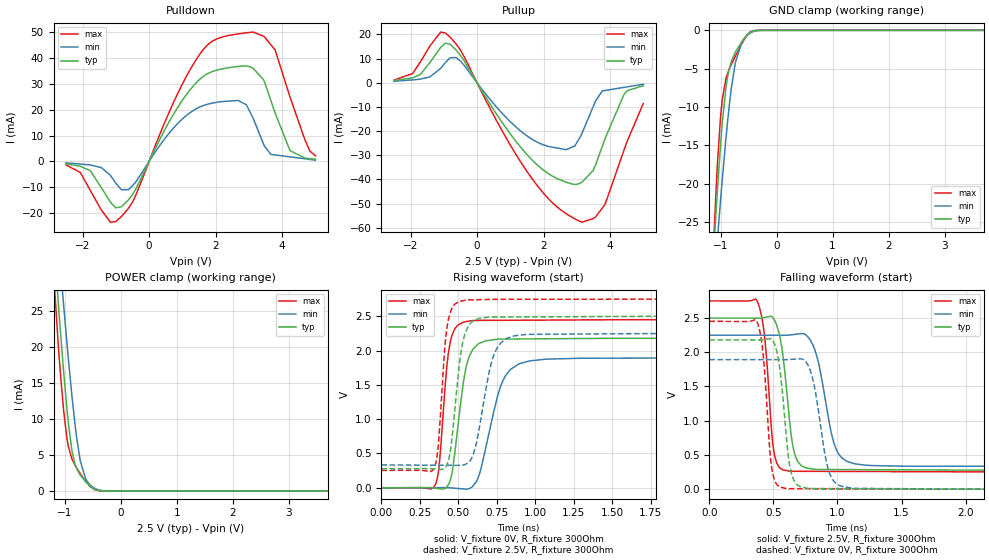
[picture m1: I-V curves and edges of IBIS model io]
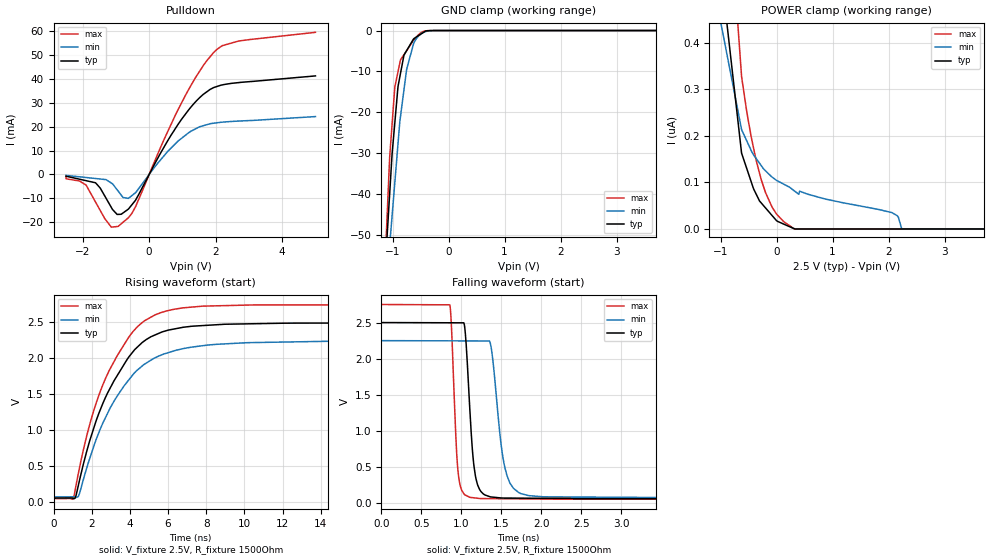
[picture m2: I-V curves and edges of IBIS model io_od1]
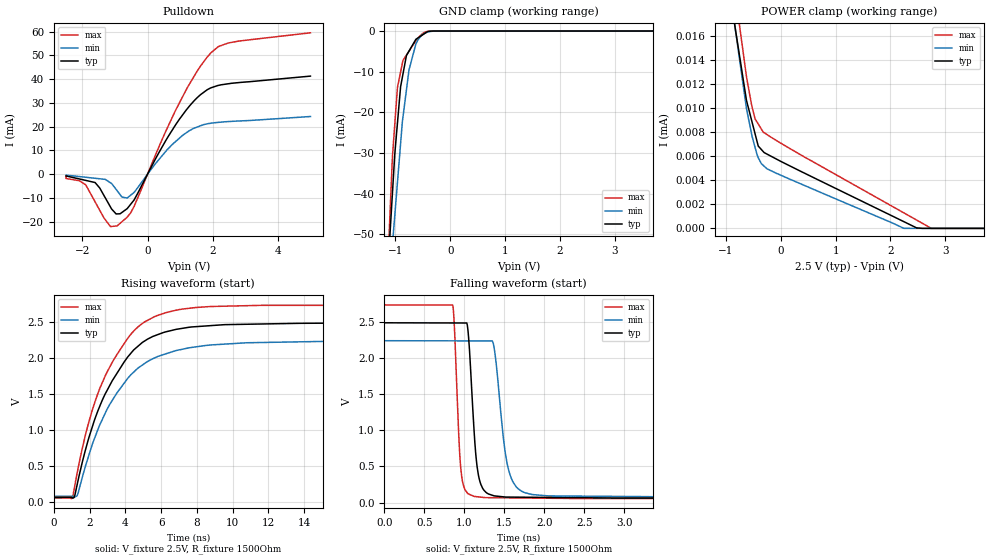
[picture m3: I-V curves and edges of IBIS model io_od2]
| Texas Instruments Incorporated
| DS250DF230 25 Gbps Multi-Rate 2-Channel Retimer
[IBIS Ver]   4.1
[File name]   ds250df230.ibs
[File Rev]   1.0
[Date]   04/26/2018
[Source]
| Texas Instruments Incorporated.
| Analog-eLab Design Center, HPA
| 12500 TI Blvd
| Dallas, TX -75243
[Notes]   Revision History:
| Rev 1.0: 04/26/2018
| - Initial version of the model.
| - Model generated from simulations in SPECTRE.
| - Model matched to SPICE simulation.
| - C_comp although listed in numerical order of value are
|   obtained from varying PVT conditions. For PVT conditions for
|   each specific value refer the buffer description under
|   respective [Model]. IBIS model user is responsible for using
|   appropriate C_comp to simulate for Signal Integrity.
| - Notes regarding non-monotonicity of various models
|   have been reviewed and considered minor and can be ignored.
[Disclaimer]
| This model is designed as an aid for customers of Texas Instruments.
| TI and its licensors and suppliers make no warranties, either expressed
| or implied, with respect to this  model, including the warranties of
| merchantability or fitness for a particular purpose. The model is
| provided solely on an "as is" basis. The entire risk as to its quality
| and performance is with the customer.
| This model is subject to change without notice. Texas Instruments
| Incorporated is not responsible for updating tDP83869his model.
[Copyright]
(C) Copyright 2018 Texas Instruments Incorporated.All rights reserved.
|  Component DS250DF230ZLS 36-pin BGA Package
|  Part # DS250DF230ZLS
[Component]   DS250DF230ZLS
[Manufacturer]  TI
[Package]   |36-pin BGA
|   typ   min   max
R_pkg   0.05   0.04   0.06
L_pkg   1.0nH   0.8nH   1.2nH
C_pkg   0.2pF   0.16pF   0.24pF
[Pin]  signal_name   model_name   R_pin   L_pin   C_pin
A1   RX1N   nc   NA   NA   NA
A2   RX1P   nc   NA   NA   NA
A3   GND   gnd   NA   NA   NA
A4   GND   gnd   NA   NA   NA
A5   RX0N   nc   NA   NA   NA
A6   RX0P   nc   NA   NA   NA
B1   GND   gnd   NA   NA   NA
B2   GND   gnd   NA   NA   NA
B3   INT_N/RCK1   io_od2   NA   NA   NA
B4   ADDR1   io   NA   NA   NA
B5   GND   gnd   NA   NA   NA
B6   GND   gnd   NA   NA   NA
C1   ADDR0   io   NA   NA   NA
C2   SDC   io_od1   NA   NA   NA
C3   VDD   power   NA   NA   NA
C4   VDD   power   NA   NA   NA
C5   TEST0/RCK0   io   NA   NA   NA
C6   EN_SMB   io   NA   NA   NA
D1   CAL_CLK_OUT   io   NA   NA   NA
D2   SDA   io_od1   NA   NA   NA
D3   VDD   power   NA   NA   NA
D4   VDD   power   NA   NA   NA
D5   THR/TEST1   io   NA   NA   NA
D6   CAL_CLK_IN   io   NA   NA   NA
E1   GND   gnd   NA   NA   NA
E2   GND   gnd   NA   NA   NA
E3   ALL_DONE_N   io   NA   NA   NA
E4   READ_EN_N   io   NA   NA   NA
E5   GND   gnd   NA   NA   NA
E6   GND   gnd   NA   NA   NA
F1   TX1N   nc   NA   NA   NA
F2   TX1P   nc   NA   NA   NA
F3   GND   gnd   NA   NA   NA
F4   GND   gnd   NA   NA   NA
F5   TX0N   nc   NA   NA   NA
F6   TX0P   nc   NA   NA   NA
| Models and submodels in the file (3): io (I/O), io_od1 (I/O_open_drain), io_od2 (I/O_open_drain)
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|   io Model
[Model]   io
Model_type   I/O
Polarity   Non-Inverting
Enable   Active-High
Vinl = 0.75
Vinh = 1.75
Vmeas = 1.25
Vref = 0
Cref = 20pF
Rref = 100000
|   typ   min   max
C_comp   0.424pF   0.417pF   0.432pF
| Where Nom  PVT is Nominal Process, 2.5V,  27C
|   Fast PVT is Strong Process,  2.75V, -40C
|   Slow PVT is Weak Process,   2.25V, 125C
[Model spec]
|subparameter
Vinl   0.75   0.675   0.825
Vinh   1.75   1.575   1.925
[Voltage Range]   2.5   2.25   2.75
|Junction Temperature
[Temperature Range]   27   125   -40
[Pullup Reference]   2.5   2.25   2.75
[Pulldown Reference]   -0   -0   0
[Power Clamp Reference]   2.5   2.25   2.75
[GND Clamp Reference]   0   0   0
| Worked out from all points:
|   slope of the pulldown table from 0 to 0.375 V, typ, clamps not added: 38 ohm
|   slope of the pullup table from 0 to 0.375 V, typ, clamps not added: 44.3 ohm
|   GND clamp passes 1 mA (typ) near -0.57 V on its own axis
|   POWER clamp passes 1 mA (typ) near -0.59 V on its own axis
|   falling waveform, V_fixture 2.5V, R_fixture 300Ohm: 20-80 % time 77.4ps typ, 117ps min, 60.5ps max; typ from 2.5 V to 0.277 V
|   rising waveform, V_fixture 0V, R_fixture 300Ohm: 20-80 % time 76.3ps typ, 123ps min, 53.2ps max; typ from 0 V to 2.18 V
|   rising waveform, V_fixture 2.5V, R_fixture 300Ohm: 20-80 % time 64.1ps typ, 96.8ps min, 47.1ps max; typ from 0.277 V to 2.5 V
|   falling waveform, V_fixture 0V, R_fixture 300Ohm: 20-80 % time 68.6ps typ, 97.8ps min, 55.2ps max; typ from 2.18 V to 0 V
[Pulldown]
|   Voltage   I(typ)   I(min)   I(max)
-2.5V     -964.9uA   -603.2uA   -1.38mA
-1.768V   -3.62mA    -1.388mA   -11.28mA
-1.003V   -17.97mA   -8.392mA   -23.3mA
-624.7mV  -14.94mA   -10.93mA   -18.21mA
695.3mV   17.39mA    12.33mA    21.7mA
1.528V    31.81mA    21.06mA    41.53mA
2.674V    36.69mA    23.55mA    49.28mA
3.128V    35.98mA    16.64mA    49.99mA
3.441V    31.54mA    6.672mA    48.39mA
3.788V    18.72mA    2.485mA    43.11mA
4.236V    4.143mA    1.738mA    24.84mA
5V        859.4uA    467.6uA    2.18mA
[GND Clamp]
|   Voltage   I(typ)   I(min)   I(max)
-2.5V     -239.4mA   -184mA     -359.8mA
-1.117V   -28.23mA   -33.1mA    -26.6mA
-1.059V   -21.15mA   -27.51mA   -17.71mA
-1.001V   -14.99mA   -22.22mA   -11.36mA
-968.2mV  -11.98mA   -19.33mA   -8.953mA
-904.5mV  -7.528mA   -14.12mA   -6.318mA
-836.2mV  -4.76mA    -9.28mA    -4.916mA
-806.2mV  -4.018mA   -7.474mA   -4.437mA
-735.7mV  -2.835mA   -4.198mA   -3.371mA
-624.7mV  -1.521mA   -1.63mA    -1.801mA
-444mV    -158.1uA   -249.7uA   -122.4uA
5V        0A         0A         0A
[Pullup]
|   Voltage   I(typ)   I(min)   I(max)
-2.5V     922.1uA    637.7uA    1.129mA
-1.705V   3.433mA    1.524mA    8.617mA
-954.7mV  16.35mA    8.33mA     20.62mA
-624.7mV  13.46mA    10.43mA    15.97mA
827.3mV   -17.87mA   -13.69mA   -21.67mA
1.751V    -33.22mA   -24.13mA   -41.47mA
2.68V     -41.09mA   -27.66mA   -54.15mA
3.153V    -41.13mA   -20.95mA   -57.66mA
3.491V    -36.26mA   -9.895mA   -56.17mA
3.85V     -23.06mA   -3.168mA   -50.26mA
4.42V     -4.767mA   -1.901mA   -27.78mA
5V        -1.206mA   -613.2uA   -8.545mA
[POWER Clamp]
|   Voltage   I(typ)   I(min)   I(max)
-2.5V     192mA      180.5mA    206mA
-1.28V    44.23mA    50.97mA    39.96mA
-1.118V   26.4mA     35.01mA    20.59mA
-1.078V   22.28mA    31.22mA    16.44mA
-1.021V   16.63mA    25.86mA    11.26mA
-939.7mV  9.743mA    18.71mA    6.308mA
-871.5mV  5.595mA    13.18mA    4.431mA
-787.5mV  3.075mA    7.406mA    3.203mA
-723mV    2.193mA    4.19mA     2.403mA
-624.7mV  1.26mA     1.658mA    1.333mA
-459.7mV  230.6uA    349.9uA    179.5uA
5V        0A         0A         0A
[Ramp]
R_load = 300
|   typ   min   max
dV/dt_r   1.30805/7.61318e-11   1.1354/1.22987e-10   1.47061/5.31016e-11
dV/dt_f   1.33347/7.72413e-11   1.15027/1.16161e-10   1.49815/6.04416e-11
[Falling Waveform]
V_fixture = 2.5V
V_fixture_min = 2.25V
V_fixture_max = 2.75V
R_fixture = 300Ohm
C_fixture = 0F
|   Time   V(typ)   V(min)   V(max)
0s        2.5V       2.25V      2.75V
375ps     2.499V     2.249V     2.742V
431.3ps   2.509V     2.249V     2.228V
506.6ps   2.475V     2.249V     520mV
623.8ps   1.046V     2.251V     263.2mV
722.7ps   337.3mV    2.274V     260.8mV
825.2ps   289.4mV    2.025V     260.2mV
993.9ps   286.5mV    566mV      259.1mV
1.219ns   284.7mV    350.2mV    257.8mV
14ns      277.3mV    332.7mV    252.9mV
[Rising Waveform]
V_fixture = 0V
V_fixture_min = 0V
V_fixture_max = 0V
R_fixture = 300Ohm
C_fixture = 0F
|   Time   V(typ)   V(min)   V(max)
0s        7.313uV    14.08uV    4.029uV
349.1ps   -6.955mV   1.034mV    41.06mV
375ps     -13.77mV   1.11mV     323.6mV
432ps     32.99mV    1.26mV     1.909V
463.5ps   284.3mV    -4.489mV   2.25V
546.9ps   1.724V     -19.69mV   2.42V
593.5ps   2.015V     23.03mV    2.437V
800.3ps   2.166V     1.611V     2.441V
1.065ns   2.171V     1.873V     2.443V
14ns      2.18V      1.892V     2.451V
[Rising Waveform]
V_fixture = 2.5V
V_fixture_min = 2.25V
V_fixture_max = 2.75V
R_fixture = 300Ohm
C_fixture = 0F
|   Time   V(typ)   V(min)   V(max)
0s        277.3mV    332.7mV    252.9mV
343.2ps   273.7mV    328.3mV    291.1mV
368.3ps   269.6mV    327.9mV    598.5mV
419.7ps   311.4mV    327.3mV    2.225V
453ps     622mV      326.8mV    2.59V
519.9ps   2.026V     328.9mV    2.721V
558.3ps   2.325V     356mV      2.736V
740.1ps   2.488V     1.988V     2.746V
942.4ps   2.49V      2.235V     2.747V
14ns      2.5V       2.25V      2.75V
[Falling Waveform]
|Gnd
V_fixture = 0V
V_fixture_min = 0V
V_fixture_max = 0V
R_fixture = 300Ohm
C_fixture = 0F
|   Time   V(typ)   V(min)   V(max)
0s        2.18V      1.892V     2.451V
372.9ps   2.179V     1.892V     2.443V
419.8ps   2.184V     1.892V     1.969V
489.4ps   2.186V     1.892V     279.9mV
601.9ps   743.2mV    1.892V     9.14mV
689ps     57.72mV    1.902V     7.25mV
803.9ps   9.562mV    1.633V     6.487mV
945.9ps   8.263mV    199.7mV    5.543mV
1.123ns   6.647mV    13.46mV    4.37mV
14ns      7.271uV    14.2uV     3.997uV
|   io_od1 Model
[Model]   io_od1
Model_type   I/O_open_drain
Polarity   Non-Inverting
Enable   Active-High
Vinl = 0.75
Vinh = 1.75
Vmeas = 1.25
Vref = 2.5
Cref = 50pF
Rref = 1500
|   typ   min   max
C_comp   0.786pF   0.768pF   0.801pF
| Where Nom  PVT is Nominal Process, 2.5V,  27C
|   Fast PVT is Strong Process,  2.75V, -40C
|   Slow PVT is Weak Process,   2.25V, 125C
[Model spec]
|subparameter
Vinl   0.75   0.675   0.825
Vinh   1.75   1.575   1.925
|0
[Voltage Range]   2.5   2.25   2.75
|Junction Temperature
[Temperature Range]   27   125   -40
[Pullup Reference]   2.5   2.25   2.75
[Pulldown Reference]   0   0   0
[Power Clamp Reference]   2.5   2.25   2.75
[GND Clamp Reference]   0   0   0
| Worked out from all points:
|   slope of the pulldown table from 0 to 0.375 V, typ, clamps not added: 38.7 ohm
|   GND clamp passes 1 mA (typ) near -0.51 V on its own axis
|   falling waveform, V_fixture 2.5V, R_fixture 1500Ohm: 20-80 % time 83.8ps typ, 131ps min, 62ps max; typ from 2.5 V to 0.06 V
|   rising waveform, V_fixture 2.5V, R_fixture 1500Ohm: 20-80 % time 2.34ns typ, 2.52ns min, 2.29ns max; typ from 0.06 V to 2.5 V
[Pulldown]
|   Voltage   I(typ)   I(min)   I(max)
-2.5V     -717uA     -384.9uA   -1.051mA
-1.897V   -2.594mA   -1.274mA   -4.43mA
-1.61V    -3.487mA   -1.697mA   -11.56mA
-1.137V   -13.79mA   -3.602mA   -22.01mA
-932.7mV  -16.69mA   -6.939mA   -21.71mA
-624.8mV  -14.48mA   -10.01mA   -18.08mA
-409.2mV  -10.77mA   -7.614mA   -13.48mA
979.9mV   23.15mA    15.15mA    30.04mA
1.515V    32.06mA    19.93mA    43.08mA
1.942V    36.31mA    21.41mA    50.99mA
2.692V    38.38mA    22.3mA     55.75mA
5V        41.17mA    24.18mA    59.38mA
[GND Clamp]
|   Voltage   I(typ)   I(min)   I(max)
-2.5V     -466.4mA   -355mA     -685.4mA
-1.143V   -60.2mA    -67.61mA   -59.4mA
-1.053V   -40.02mA   -52.63mA   -31.06mA
-1.01V    -30.17mA   -45.31mA   -22.86mA
-961.2mV  -22.6mA    -37.22mA   -13.84mA
-903.9mV  -13.68mA   -27.64mA   -10.06mA
-871.6mV  -11.34mA   -22.27mA   -7.925mA
-798.2mV  -6.031mA   -14.53mA   -5.918mA
-750.8mV  -4.935mA   -9.534mA   -4.941mA
-624.8mV  -2.02mA    -3.15mA    -2.341mA
-462.5mV  -576.6uA   -539uA     -281.7uA
5V        0A         0A         0A
[POWER Clamp]
|   Voltage   I(typ)   I(min)   I(max)
-2.5V     31.87uA    37.47uA    31.39uA
-1.114V   684.1nA    516.6nA    1.151uA
-624.9mV  163.1nA    213.7nA    328.2nA
-518mV    124.8nA    185.7nA    242.2nA
-365mV    75.08nA    151.6nA    147.8nA
-197mV    45.21nA    125nA      78.19nA
17.09mV   16.41nA    103.3nA    29.75nA
318.7mV   503pA      81.74nA    0A
2.063V    0A         34.99nA    0A
2.175V    0A         25.26nA    0A
2.236V    0A         0A         0A
5V        0A         0A         0A
[Ramp]
R_load = 1500
|   typ   min   max
dV/dt_r   1.46371/2.34371e-09   1.30382/2.52203e-09   1.61805/2.28675e-09
dV/dt_f   1.46371/8.35285e-11   1.30382/1.30915e-10   1.61805/6.18717e-11
[Falling Waveform]
V_fixture = 2.5V
V_fixture_min = 2.25V
V_fixture_max = 2.75V
R_fixture = 1500Ohm
C_fixture = 0F
|   Time   V(typ)   V(min)   V(max)
0s        2.5V       2.25V      2.75V
855.4ps   2.497V     2.247V     2.745V
949.6ps   2.497V     2.247V     557.4mV
1.031ns   2.496V     2.246V     131.6mV
1.147ns   633.2mV    2.246V     75.5mV
1.232ns   183.8mV    2.246V     63.88mV
1.371ns   86.09mV    2.168V     62.68mV
1.569ns   70.71mV    389.4mV    60.98mV
1.842ns   68.76mV    104.7mV    58.62mV
20ns      60.43mV    76.8mV     53.19mV
[Rising Waveform]
V_fixture = 2.5V
V_fixture_min = 2.25V
V_fixture_max = 2.75V
R_fixture = 1500Ohm
C_fixture = 0F
|   Time   V(typ)   V(min)   V(max)
0s        60.43mV    76.8mV     53.19mV
1.036ns   55.1mV     77.44mV    50.91mV
1.301ns   236mV      82.92mV    401.7mV
2.244ns   1.143V     881.4mV    1.389V
2.906ns   1.558V     1.278V     1.827V
3.933ns   2.016V     1.699V     2.292V
5.102ns   2.302V     1.976V     2.574V
6.776ns   2.433V     2.136V     2.703V
15.43ns   2.492V     2.24V      2.744V
90ns      2.5V       2.25V      2.75V
|   io_od2 Model
[Model]   io_od2
Model_type   I/O_open_drain
Polarity   Non-Inverting
Enable   Active-High
Vinl = 0.75
Vinh = 1.75
Vmeas = 1.25
Vref = 2.5
Cref = 50pF
Rref = 1500
|   typ   min   max
C_comp   0.783pF   0.772pF   0.797pF
| Where Nom  PVT is Nominal Process, 2.5V,  27C
|   Fast PVT is Strong Process,  2.75V, -40C
|   Slow PVT is Weak Process,   2.25V, 125C
[Model spec]
|subparameter
Vinl   0.75   0.675   0.825
Vinh   1.75   1.575   1.925
[Voltage Range]   2.5   2.25   2.75
|Junction Temperature
[Temperature Range]   27   125   -40
[Pullup Reference]   2.5   2.25   2.75
[Pulldown Reference]   0   -0   0
[Power Clamp Reference]   2.5   2.25   2.75
[GND Clamp Reference]   0   0   0
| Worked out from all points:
|   slope of the pulldown table from 0 to 0.375 V, typ, clamps not added: 38.7 ohm
|   GND clamp passes 1 mA (typ) near -0.51 V on its own axis
|   falling waveform, V_fixture 2.5V, R_fixture 1500Ohm: 20-80 % time 84.2ps typ, 132ps min, 62.5ps max; typ from 2.49 V to 0.06 V
|   rising waveform, V_fixture 2.5V, R_fixture 1500Ohm: 20-80 % time 2.52ns typ, 2.71ns min, 2.48ns max; typ from 0.06 V to 2.49 V
[Pulldown]
|   Voltage   I(typ)   I(min)   I(max)
-2.5V     -717uA     -384.9uA   -1.051mA
-1.897V   -2.594mA   -1.274mA   -4.43mA
-1.61V    -3.487mA   -1.697mA   -11.56mA
-1.137V   -13.79mA   -3.602mA   -22.01mA
-932.7mV  -16.69mA   -6.939mA   -21.71mA
-624.8mV  -14.48mA   -10.01mA   -18.08mA
-409.2mV  -10.77mA   -7.614mA   -13.48mA
976.4mV   23.08mA    15.12mA    29.91mA
1.512V    32.01mA    19.78mA    43.08mA
1.944V    36.32mA    21.43mA    51.03mA
2.474V    38.02mA    22.13mA    55.16mA
5V        41.25mA    24.26mA    59.45mA
[GND Clamp]
|   Voltage   I(typ)   I(min)   I(max)
-2.5V     -466.4mA   -355mA     -685.4mA
-1.143V   -60.21mA   -67.62mA   -59.41mA
-1.053V   -40.03mA   -52.64mA   -31.07mA
-1.01V    -30.18mA   -45.32mA   -22.87mA
-961.2mV  -22.61mA   -37.22mA   -13.85mA
-903.9mV  -13.68mA   -27.65mA   -10.07mA
-871.6mV  -11.34mA   -22.27mA   -7.932mA
-798.2mV  -6.037mA   -14.53mA   -5.924mA
-750.8mV  -4.94mA    -9.54mA    -4.947mA
-624.8mV  -2.024mA   -3.153mA   -2.345mA
-462.5mV  -578.4uA   -540.9uA   -283.3uA
5V        0A         0A         0A
[POWER Clamp]
|   Voltage   I(typ)   I(min)   I(max)
-2.5V     107.4uA    112.3uA    112.8uA
-1.256V   29.16uA    30.44uA    33.84uA
-624.9mV  10.65uA    9.969uA    12.63uA
-518mV    8.754uA    7.579uA    10.01uA
-468.5mV  7.877uA    6.747uA    9.112uA
-411.1mV  6.859uA    5.891uA    8.687uA
-320mV    6.391uA    5.244uA    8.012uA
-90.06mV  5.792uA    4.604uA    7.34uA
2.245V    557.6nA    1.369nA    1.287uA
2.475V    42.43nA    0A         696.2nA
2.744V    0A         0A         1.776nA
5V        0A         0A         0A
[Ramp]
R_load = 1500
|   typ   min   max
dV/dt_r   1.45872/2.51535e-09   1.29995/2.69506e-09   1.61172/2.47441e-09
dV/dt_f   1.45872/8.416e-11   1.29995/1.3217e-10   1.61172/6.22816e-11
[Falling Waveform]
V_fixture = 2.5V
V_fixture_min = 2.25V
V_fixture_max = 2.75V
R_fixture = 1500Ohm
C_fixture = 0F
|   Time   V(typ)   V(min)   V(max)
0s        2.492V     2.243V     2.739V
854.9ps   2.489V     2.241V     2.737V
966.6ps   2.489V     2.241V     371.7mV
1.045ns   2.4V       2.241V     124.6mV
1.125ns   954.6mV    2.241V     84.76mV
1.2ns     277.5mV    2.241V     75.58mV
1.362ns   96.89mV    2.209V     67.01mV
1.554ns   75.52mV    456.5mV    64.93mV
1.848ns   72.67mV    110.9mV    61.74mV
20ns      60.43mV    76.79mV    53.19mV
[Rising Waveform]
V_fixture = 2.5V
V_fixture_min = 2.25V
V_fixture_max = 2.75V
R_fixture = 1500Ohm
C_fixture = 0F
|   Time   V(typ)   V(min)   V(max)
0s        60.43mV    76.79mV    53.19mV
1.036ns   55mV       77.43mV    50.86mV
1.301ns   234.2mV    83.12mV    395.7mV
2.312ns   1.164V     905.5mV    1.401V
3.036ns   1.577V     1.314V     1.832V
4.045ns   1.985V     1.688V     2.244V
5.066ns   2.236V     1.923V     2.502V
7.175ns   2.413V     2.122V     2.681V
16.53ns   2.485V     2.235V     2.734V
90ns      2.492V     2.243V     2.739V
